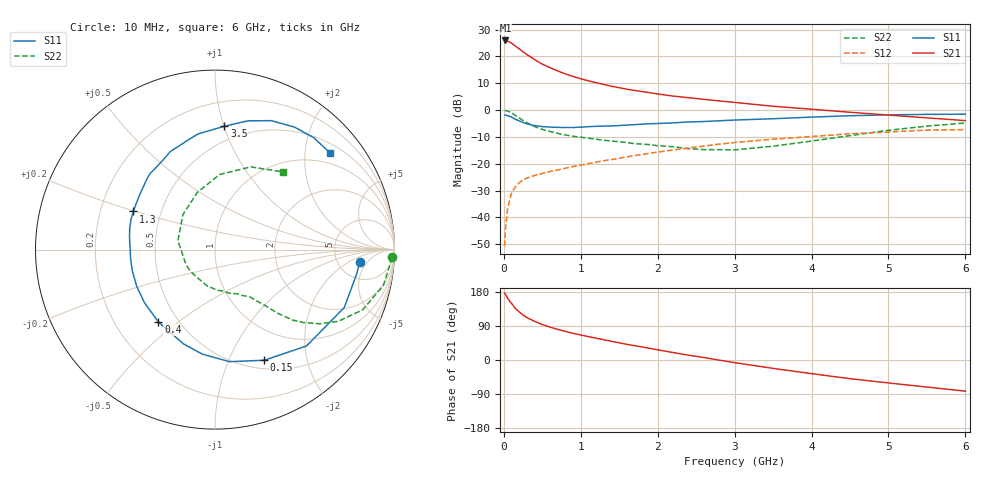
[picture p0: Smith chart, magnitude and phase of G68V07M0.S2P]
! SIEMENS Small Signal Semiconductors
! BFG193
! Si NPN RF Bipolar Junction Transistor in SOT223
! VCE = 8 V  IC = 7 mA
! Common Emitter S-Parameters:  August  1996
# GHz  S  MA  R  50
!  f  S11  S21  S12  S22
! GHz  MAG  ANG  MAG  ANG  MAG  ANG  MAG  ANG
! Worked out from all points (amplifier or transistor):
!   36 points, 10 MHz to 6 GHz, reference 50 ohm
!   highest |S21| = 26.0 dB at 20 MHz (marker M1)
!   |S21| within 3 dB of that: start of sweep to 193.8 MHz
!   unconditionally stable (mu >= 1): 1.042 GHz to 2.53 GHz
!   at 250 MHz: K = 0.41, MSG = 23.9 dB, |S12| = -26.0 dB
!   at 1.4 GHz: K = 1.08, MAG = 12.0 dB, |S12| = -18.5 dB
!   at 6 GHz: K = 0.86, MSG = 1.7 dB, |S12| = -7.3 dB
!   S11 on the Smith chart (normalised r, x): 10 MHz: 8.16, -3.27; 150 MHz: 0.60, -1.36; 400 MHz: 0.39, -0.43; 1.3 GHz: 0.35, +0.20; 3.5 GHz: 0.38, +1.00; 6 GHz: 0.71, +2.57
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0.01  0.8092 -4.9  19.8 176.2  0.0029 86.4  0.9855 -2.5
0.02  0.8009 -9.8  19.86 173.7  0.006 89.7  0.9781 -4.9
0.05  0.7894 -24.1  19.25 162.7  0.015 77.0  0.9593 -12.0
0.1  0.7405 -46.5  17.68 149.4  0.0283 68.3  0.8883 -22.2
0.15  0.6747 -66.0  15.62 135.9  0.0372 59.4  0.7945 -30.2
0.2  0.6298 -82.6  13.85 126.8  0.0442 55.0  0.7152 -35.3
0.25  0.5864 -97.0  12.21 118.4  0.0501 50.4  0.6388 -39.5
0.3  0.5534 -108.7  10.84 111.9  0.054 48.3  0.583 -42.3
0.4  0.512 -128.0  8.714 102.0  0.0605 45.5  0.4928 -45.6
0.5  0.4918 -143.1  7.184 93.4  0.0657 44.1  0.4361 -47.4
0.6  0.4819 -154.8  6.167 86.8  0.0715 44.2  0.3979 -49.1
0.7  0.4758 -165.2  5.37 80.8  0.0764 44.7  0.3679 -51.0
0.9  0.4734 178.8  4.23 70.5  0.0887 44.4  0.3251 -53.8
1.1  0.49 166.0  3.509 61.7  0.1004 44.7  0.2983 -59.1
1.3  0.5018 154.9  2.999 53.4  0.1139 43.9  0.2735 -63.9
1.6  0.5253 141.0  2.447 41.3  0.1344 41.6  0.2475 -74.5
2.2  0.5767 120.2  1.824 19.7  0.1805 34.4  0.2073 -101.8
2.8  0.6315 103.1  1.481 -0.3  0.2316 24.3  0.1829 -139.9
3.5  0.6895 85.6  1.179 -22.1  0.2863 9.2  0.2123 166.7
4.5  0.7841 66.4  0.91 -49.3  0.3622 -10.7  0.3338 107.2
5.5  0.8317 48.5  0.716 -71.4  0.4235 -35.9  0.502 66.6
6  0.8374 40.0  0.636 -82.3  0.4321 -50.5  0.5741 49.0
